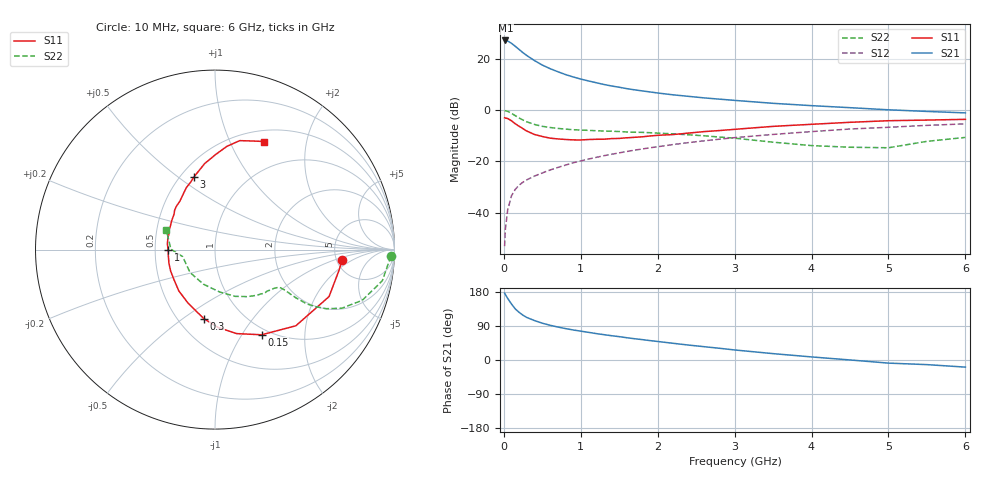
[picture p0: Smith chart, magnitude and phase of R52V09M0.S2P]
! SIEMENS Small Signal Semiconductors
! BFR183
! Si NPN RF Bipolar Junction Transistor in SOT23
! VCE = 2 V  IC = 9 mA
! Common Emitter S-Parameters:  May  1996
# GHz  S  MA  R  50
!  f  S11  S21  S12  S22
! GHz  MAG  ANG  MAG  ANG  MAG  ANG  MAG  ANG
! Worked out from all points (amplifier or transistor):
!   36 points, 10 MHz to 6 GHz, reference 50 ohm
!   highest |S21| = 27.2 dB at 20 MHz (marker M1)
!   |S21| within 3 dB of that: start of sweep to 177.5 MHz
!   unconditionally stable (mu >= 1): 776.4 MHz to 2.514 GHz
!   at 250 MHz: K = 0.60, MSG = 25.3 dB, |S12| = -28.1 dB
!   at 1.4 GHz: K = 1.06, MAG = 11.9 dB, |S12| = -17.2 dB
!   at 6 GHz: K = 0.90, MSG = 2.1 dB, |S12| = -5.3 dB
!   S11 on the Smith chart (normalised r, x): 10 MHz: 5.59, -1.31; 150 MHz: 0.91, -1.23; 300 MHz: 0.66, -0.60; 1 GHz: 0.59, -0.00; 3 GHz: 0.58, +0.58; 6 GHz: 0.63, +1.35
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0.01  0.7105 -4.7  22.93 176.5  0.0022 88.4  0.9817 -2.1
0.02  0.701 -9.3  23.04 172.6  0.0047 87.9  0.9701 -4.3
0.05  0.6872 -22.4  22.49 162.5  0.0113 79.7  0.948 -10.6
0.1  0.6189 -43.3  20.21 147.6  0.0213 72.3  0.8676 -19.0
0.15  0.541 -61.3  17.65 134.5  0.0285 65.7  0.7785 -24.8
0.2  0.4831 -75.6  15.28 125.5  0.0344 63.2  0.7014 -28.0
0.25  0.4337 -87.8  13.24 118.0  0.0393 61.0  0.6398 -29.7
0.3  0.39 -99.1  11.65 112.1  0.0437 61.3  0.5919 -30.6
0.4  0.3342 -116.6  9.289 103.9  0.0517 61.1  0.5249 -30.8
0.5  0.306 -131.2  7.609 97.1  0.0593 61.9  0.4835 -30.5
0.6  0.2841 -143.2  6.486 91.7  0.0677 62.6  0.4589 -30.2
0.7  0.2745 -154.2  5.653 87.1  0.0758 63.6  0.4407 -30.1
0.8  0.2676 -163.4  4.977 83.0  0.0843 63.5  0.4262 -30.2
1  0.2616 -179.6  4.055 76.1  0.1019 64.1  0.4088 -30.9
1.1  0.267 173.3  3.727 73.0  0.1108 64.1  0.403 -32.0
1.6  0.2888 147.0  2.633 58.7  0.156 61.9  0.3749 -37.6
2.2  0.3337 125.8  1.995 44.1  0.2128 57.3  0.3448 -47.6
3  0.4223 106.0  1.554 26.5  0.2906 48.8  0.2836 -66.7
3.5  0.4824 96.9  1.361 16.8  0.3357 42.6  0.2368 -84.1
4.5  0.5793 83.4  1.119 0.1  0.4284 30.1  0.1886 -137.7
5.5  0.6406 70.8  0.945 -12.2  0.5049 18.0  0.2459 179.4
6  0.6618 65.5  0.885 -18.8  0.5403 10.2  0.2936 157.7
